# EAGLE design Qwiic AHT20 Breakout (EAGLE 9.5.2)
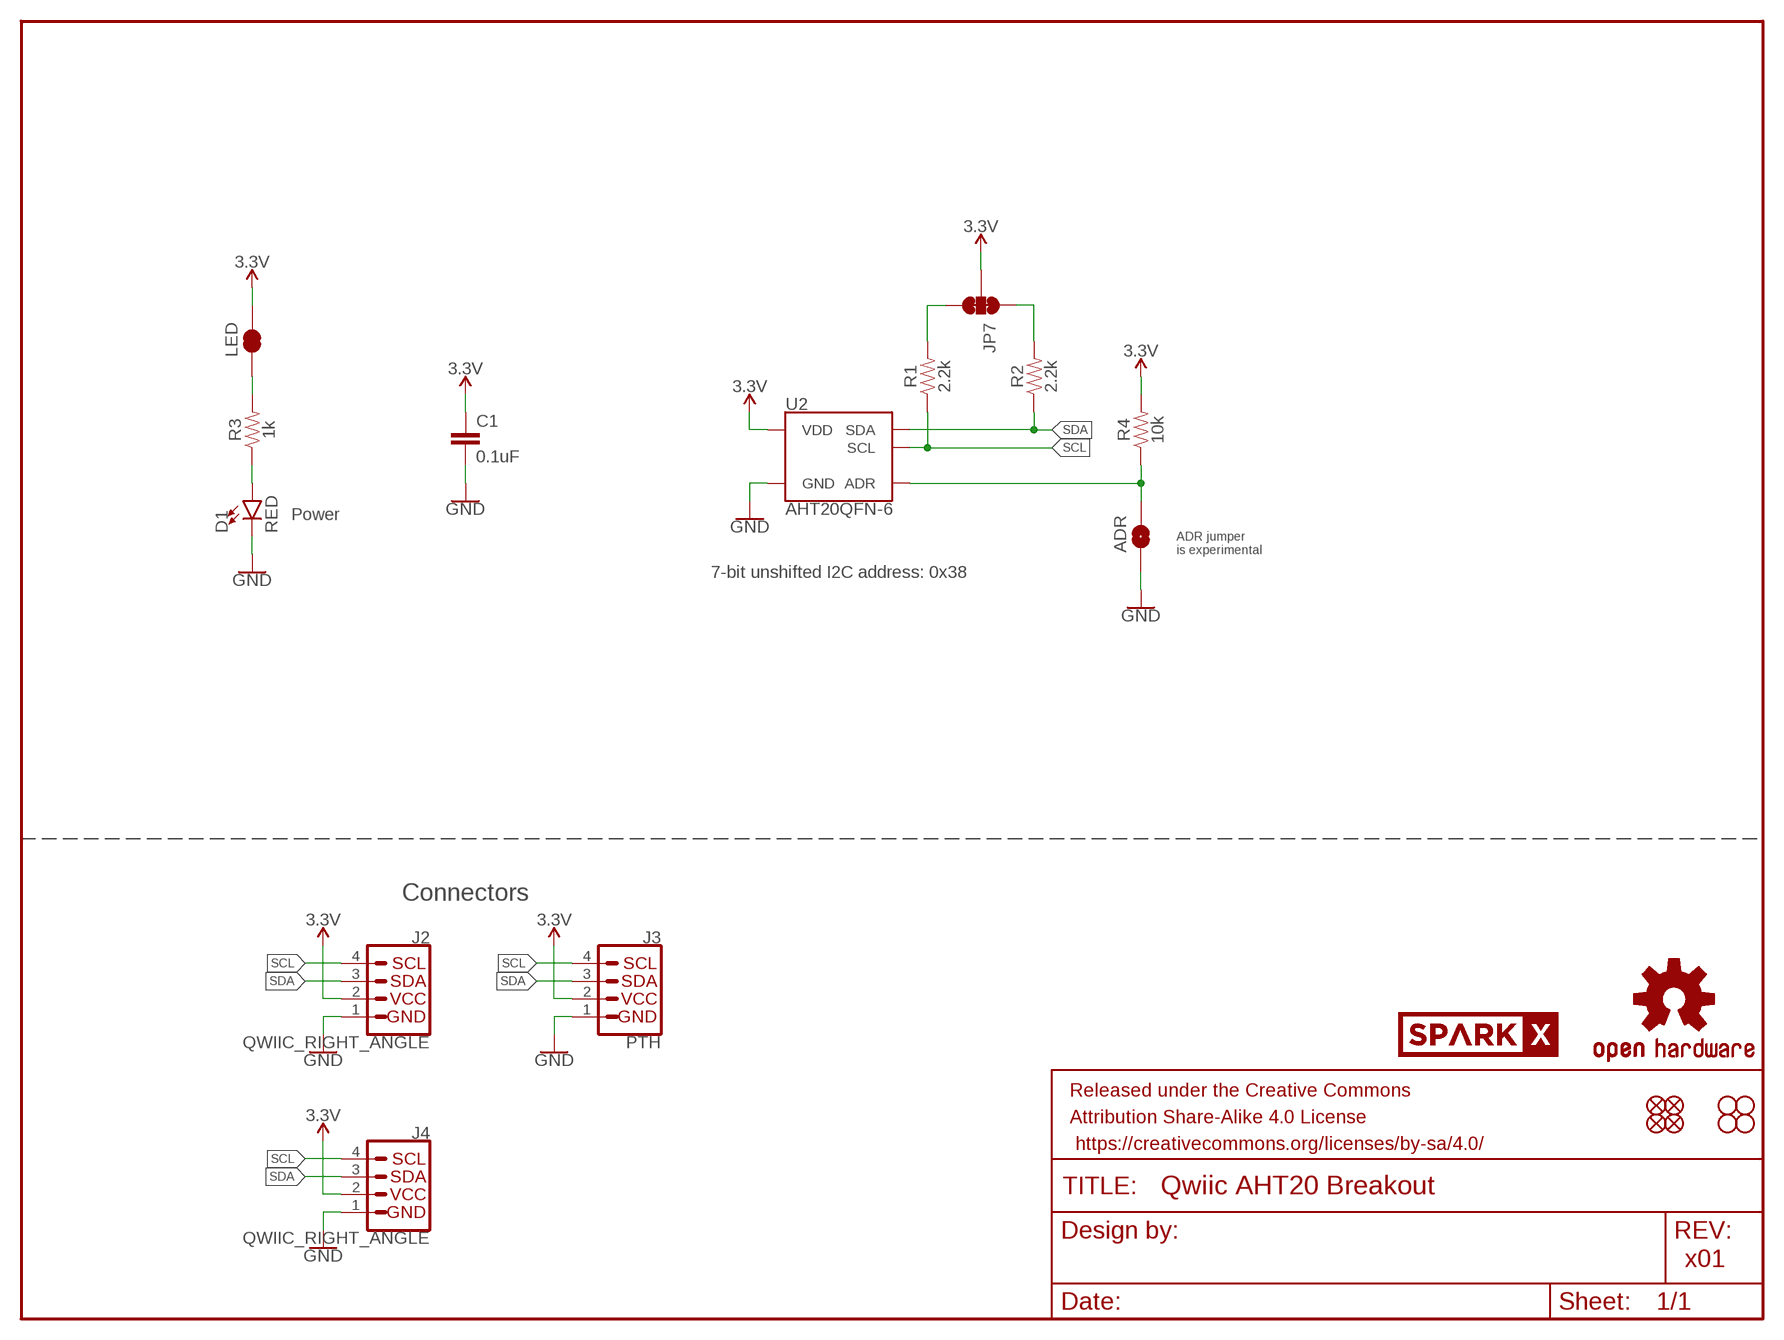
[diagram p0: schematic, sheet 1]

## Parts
ADR  JUMPER-SMT_2_NO_SILK  [SMT-JUMPER_2_NO_SILK]
C1  0.1uF  0.1UF-0603-25V-(+80/-20%)  [0603]
D1  RED  LED-RED0603  [LED-0603]
FRAME1  FRAME-LETTER  [CREATIVE_COMMONS]
J2  QWIIC_RIGHT_ANGLE  QWIIC_CONNECTORJS-1MM  [JST04_1MM_RA]
J3  PTH  I2C_STANDARD_NO_SILK  [1X04_NO_SILK]
J4  QWIIC_RIGHT_ANGLE  QWIIC_CONNECTORJS-1MM  [JST04_1MM_RA]
JP1  FIDUCIAL1X2  [FIDUCIAL-1X2]
JP2  FIDUCIAL1X2  [FIDUCIAL-1X2]
JP3  STAND-OFF  [STAND-OFF]
JP4  STAND-OFF  [STAND-OFF]
JP5  FIDUCIAL1X2  [FIDUCIAL-1X2]
JP6  FIDUCIAL1X2  [FIDUCIAL-1X2]
JP7  JUMPER-SMT_3_2-NC_TRACE_SILK  [SMT-JUMPER_3_2-NC_TRACE_SILK]
JP8  STAND-OFF  [STAND-OFF]
JP9  STAND-OFF  [STAND-OFF]
LED  JUMPER-SMT_2_NC_TRACE_SILK  [SMT-JUMPER_2_NC_TRACE_SILK]
LOGO1  OSHW-LOGOMINI  [OSHW-LOGO-MINI]
R1  2.2k  2.2KOHM-0603-1/10W-1%  [0603]
R2  2.2k  2.2KOHM-0603-1/10W-1%  [0603]
R3  1k  1KOHM-0603-1/10W-1%  [0603]
R4  10k  10KOHM-0603-1/10W-1%  [0603]
U2  AHT20QFN-6  [QFN-6]
U$1  SPARKX-LOGO4  [SPARKX-MEDIUM]
U$2  SPARKX-LOGO4  [SPARKX-MEDIUM]

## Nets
3.3V: C1.1 J2.2 J3.2(VCC) J4.2 JP7.2 LED.2 R4.2 U2.VDD
GND: ADR.1 C1.2 D1.C J2.1 J3.1(GND) J4.1 U2.GND
N$1: JP7.3 R1.2
N$2: JP7.1 R2.2
N$3: D1.A R3.1
N$4: LED.1 R3.2
N$5: ADR.2 R4.1 U2.ADR
SCL: J2.4 J3.4(SCL) J4.4 R1.1 U2.SCL
SDA: J2.3 J3.3(SDA) J4.3 R2.1 U2.SDA

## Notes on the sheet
- Power
- ADR jumper
  is experimental
- 7-bit unshifted I2C address: 0x38
- Connectors
- x01

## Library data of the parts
ADR = SparkFun-Jumpers:JUMPER-SMT_2_NO: Normally open jumper
C1 = SparkFun-Capacitors:0.1UF: 0.1µF ceramic capacitors; PROD_ID: CAP-00810
D1 = SparkFun-LED:LED-RED: Red SMD LED; PROD_ID: DIO-00819
FRAME1 = SparkFun-Aesthetics:FRAME-LETTER: Schematic Frame - Letter
J2 J4 = SparkFun-Connectors:QWIIC_CONNECTOR: SparkFun I2C Standard Qwiic Connector An SMD 1mm pitch JST connector makes it easy and quick (get it? Qwiic?) to connect I2C devices to each other. The Qwiic system enables fast and solderless connection between popular platforms and various sensors and actuators. We carry 200mm, 100mm, 50mm, and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; PROD_ID: CONN-13694
J3 = SparkX:I2C_STANDARD: SparkFun I2C Standard Pinout Header SparkFun has standardized on a pinout for all I2C based sensor breakouts. This pinout allows I2C boards to be plugged directly into the headers on Arduino Uno compatible boards, and to be daisy chained easily. Example SparkFun Products: SparkFun Atmospheric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
JP1 JP2 JP5 JP6 = SparkFun-Aesthetics:FIDUCIAL: Fiducial Alignment Points
JP3 JP4 JP8 JP9 = SparkFun-Hardware:STAND-OFF: Stand Off
JP7 = SparkFun-Jumpers:JUMPER-SMT_3_2-NC_TRACE: Normally closed trace jumper (2 of 2 connections) This jumper has a trace between all three pads so they are normally closed (NC). Use a razor knife to open the connection(s). For best results follow the IPC guidelines for cutting traces: Cutout at least 0.063 mm (0.005 in). Remove all loose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
LED = SparkFun-Jumpers:JUMPER-SMT_2_NC_TRACE: Normally closed trace jumper
LOGO1 = SparkFun-Aesthetics:OSHW-LOGO: Open-Source Hardware (OSHW) Logo
R1 R2 = SparkFun-Resistors:2.2KOHM: 2.2kΩ resistor; PROD_ID: RES-08272
R3 = SparkFun-Resistors:1KOHM: 1kΩ resistor; PROD_ID: RES-07856
R4 = SparkFun-Resistors:10KOHM: 10kΩ resistor; PROD_ID: RES-00824
U2 = AHT20:AHT20: Aosong AHT20 I2C Humidity and Temperature Sensor The AHT20 is a low-cost, easy-to-use, highly accurate, digital humidity and temperature sensor. AHT20 is equipped with a newly designed ASIC chip, an improved MEMS semiconductor capacitive humidity sensing element and a standard on-chip temperature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; PROD_ID: IC-
U$1 U$2 = SparkX:SPARKX-LOGO

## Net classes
1 power: width 0.203 mm

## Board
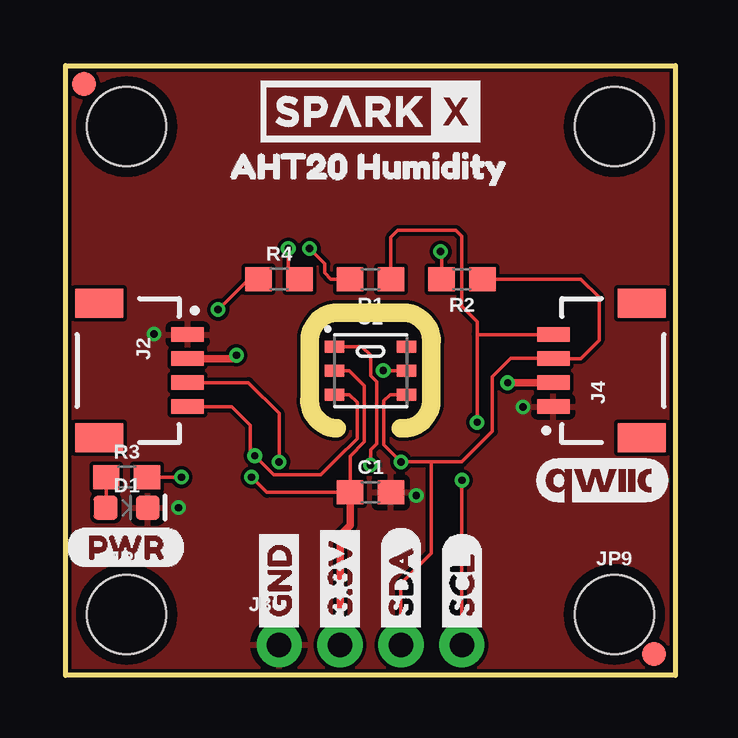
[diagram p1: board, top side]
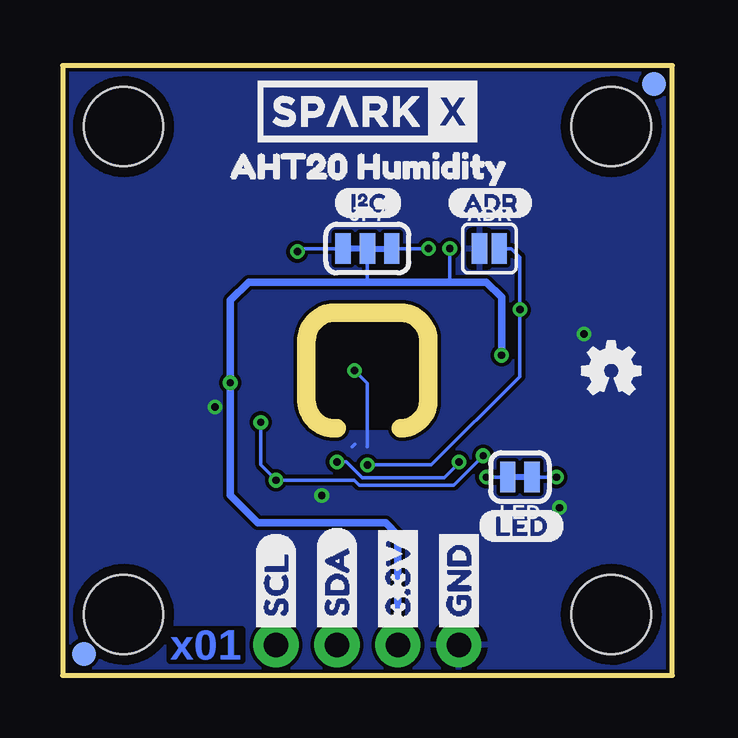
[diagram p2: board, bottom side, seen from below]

Size 25.4 x 25.4 mm. Coordinates in mm from the lower left corner, seen from the top.
Outline: 13.97,10.29 arc92 15.24,11.43 15.24,13.84 arc92 14.1,15.11 11.43,15.11 arc92 10.16,13.97 10.16,11.56 arc92 11.3,10.29
Outline: 0,0 0,25.4 25.4,25.4 25.4,0 0,0
Copper layers (1*16): Top 0.035mm / dielectric 1.5mm / Bottom 0.035mm
Design rules "SparkFun-2-layer-PCBWay-LIMIT": minimum track width 6mil, minimum drill 0.3mm, track to track 6mil, track to pad 6mil, pad to pad 6mil, via to via 6mil, smd to smd 6mil, copper to edge 6mil, drill to drill 6mil, minimum pad ring 6mil, minimum via ring 6mil, stop-mask expansion 4mil, vias tented up to drill 25mil, thermal gap 10mil

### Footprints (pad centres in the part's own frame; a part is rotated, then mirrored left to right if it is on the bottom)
SMT-JUMPER_2_NO_SILK = smd 0.635 x 1.27: 1 -0.406,0; 2 0.406,0
0603 = smd 1.1 x 1: 1 -0.85,0; 2 0.85,0
LED-0603 = smd 1 x 1: A -0.877,0; C 0.877,0
JST04_1MM_RA = smd 0.6 x 1.35: 1 -1.5,0; 2 -0.5,0; 3 0.5,0; 4 1.5,0 | smd 1.2 x 2: NC1 2.8,-3.675; NC2 -2.8,-3.675
1X04_NO_SILK = drill 1.016 pad 1.88: 1 0,0; 2 2.54,0; 3 5.08,0; 4 7.62,0
FIDUCIAL-1X2 = smd 1 x 1: 1 0,0
STAND-OFF = hole 3.302: 0,0
SMT-JUMPER_3_2-NC_TRACE_SILK = smd 0.635 x 1.27: 1 -1.016,0; 2 0,0; 3 1.016,0
SMT-JUMPER_2_NC_TRACE_SILK = smd 0.635 x 1.27: 1 -0.508,0; 2 0.508,0
QFN-6 = smd 0.8 x 0.5: ADR -1.5,1; GND 1.5,0; NC2 1.5,1; SCL -1.5,-1; SDA 1.5,-1; VDD -1.5,0

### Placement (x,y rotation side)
ADR  7.62,17.78 0 bottom
C1  12.7,7.62 0 top
D1  2.54,6.99 0 top
FRAME1  not placed on the board
J2  5.08,12.7 270 top
J3  8.89,1.27 0 top
J4  20.32,12.7 90 top
JP1  0.76,24.64 0 bottom
JP2  24.51,0.89 0 top
JP3  2.54,22.86 0 top
JP4  22.86,22.86 0 top
JP5  24.51,0.89 0 bottom
JP6  0.76,24.64 0 top
JP7  12.7,17.78 0 bottom
JP8  2.54,2.54 0 top
JP9  22.86,2.54 0 top
LED  6.35,8.26 180 bottom
LOGO1  2.54,12.7 0 bottom
R1  12.7,16.51 180 top
R2  16.51,16.51 180 top
R3  2.54,8.26 0 top
R4  8.89,16.51 0 top
U2  12.7,12.7 0 top
U$1  12.7,23.5 0 top
U$2  12.7,23.5 0 bottom
U$3  [GND1]  8.89,1.52 90 bottom
U$4  [3#3V2]  11.43,1.52 90 bottom
U$5  [SDA8]  13.97,1.52 90 bottom
U$6  [SCL9]  16.51,1.52 90 bottom
U$8  [AHT20_HUMIDITY2]  19.3,21.21 0 bottom
U$9  [I_SUPER2_C-()-03]  14.1,19.68 0 bottom
U$10  [(PWR)]  0,5.33 0 top
U$11  [QWIIC_5.5MM]  22.35,8.13 0 top
U$12  [LED_32]  8.13,6.22 0 bottom
U$13  [ADR-()-03]  9.4,19.68 0 bottom
U$14  [AHT20_HUMIDITY2]  5.97,21.21 0 top
U$18  [ORDERING_INSTRUCTIONS]  not placed on the board
U$21  [3#3V2]  11.43,1.52 90 top
U$22  [GND1]  8.89,1.52 90 top
U$26  [SCL9]  16.51,1.52 90 top
U$27  [SDA8]  13.97,1.52 90 top

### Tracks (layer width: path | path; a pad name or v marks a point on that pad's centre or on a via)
3.3V  (via drill 0.3)
  Top 0.152: U2.VDD 11.81,12.7 12.45,12.06 12.45,9.73 11.85,9.13 C1.1 8.38,7.62 v7.75,8.26 | R4.2 9.27,16.98 v9.27,17.78
  Top 0.305: J2.2 6.98,13.2 v7.11,13.34 | v18.41,12.19 J4.2 | J3.2 11.43,5.84 11.85,6.26 C1.1
  Bottom 0.152: LED.2 v7.75,8.26 | JP7.2 12.7,16.38 | v9.27,17.78 9.27,16.38
  Bottom 0.305: v7.11,13.34 7.11,15.75 7.75,16.38 9.27,16.38 12.7,16.38 17.65,16.38 18.41,15.62 v18.41,12.19 18.41,7.49 17.27,6.35 11.94,6.35 11.43,5.84 J3.2
GND  (via drill 0.3)
  Top 0.152: U2.GND v13.23,12.7
  Bottom 0.152: 13.23,9.63 13.34,9.53 | v13.23,12.7 12.7,12.17 12.7,9.53
  other vias: 14.61,7.49 19.05,11.18 4.7,6.99 3.68,14.22
  pour Bottom (isolate 0.152): 0,0 0,25.4 25.4,25.4 25.4,0
  pour Top (isolate 0.152): 0,0 0,25.4 25.4,25.4 25.4,0
N$1  (via drill 0.3)
  Top 0.152: R1.2 11.05,16.51 10.79,16.76 10.79,17.14 v10.16,17.78
  Bottom 0.152: JP7.3 v10.16,17.78
N$2  (via drill 0.3)
  Top 0.152: v15.62,17.65 15.66,17.61 R2.2
  Bottom 0.152: JP7.1 15.49,17.78 v15.62,17.65
N$3
  Top 0.152: R3.1 1.69,7.01 D1.A
N$4  (via drill 0.3)
  Top 0.152: R3.2 v4.83,8.26
  Bottom 0.152: LED.1 v4.83,8.26
N$5  (via drill 0.3)
  Top 0.152: U2.ADR 12.34,13.7 12.7,13.34 12.7,12.48 12.95,12.22 12.95,9.65 12.7,9.4 v12.7,8.76 | R4.1 7.62,16.51 v6.35,15.24
  Bottom 0.152: v12.7,8.76 10.03,8.76 6.35,12.45 v6.35,15.24 6.35,17.42 6.71,17.78 ADR.2
N$6
  cutout Bottom (isolate 0.305): 10.41,14.86 14.99,14.86 14.99,10.29 10.41,10.29
  cutout Top (isolate 0.305): 14.99,14.86 10.41,14.86 10.41,10.29 14.99,10.29
SCL  (via drill 0.3)
  Top 0.152: U2.SCL 11.82,11.7 12.14,11.38 12.14,9.86 11.3,9.02 11.29,9.02 10.63,8.36 8.67,8.36 v7.88,9.15 7.7,9.33 7.7,10.41 6.91,11.2 J2.4 | 17.14,14.22 17.14,14.73 16.51,15.37 16.51,18.29 16.26,18.54 13.84,18.54 13.55,18.25 R1.1 | 17.14,14.22 v17.14,10.54 | 17.14,14.22 17.17,14.2 J4.4 | J3.4 v16.51,8.13
  Bottom 0.152: v17.14,10.54 17.14,8.76 v16.51,8.13 13.25,8.13 13.05,7.92 9.1,7.92 v7.88,9.15
SDA  (via drill 0.3)
  Top 0.152: J2.3 7.61,12.2 8.89,10.92 v8.89,8.89 | 15.24,8.89 v13.97,8.89 13.26,9.6 13.26,9.65 13.26,10.16 13.26,11.43 13.53,11.7 U2.SDA | 15.24,8.89 16.51,8.89 17.78,10.16 17.78,12.45 18.54,13.21 J4.3 21.45,13.2 22.23,13.97 22.23,15.75 21.46,16.51 R2.1 | J3.3 13.97,3.81 15.24,5.08 15.24,8.89
  Bottom 0.152: v13.97,8.89 13.58,8.89 12.92,8.23 9.5,8.23 8.89,8.84 v8.89,8.89

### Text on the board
Bottom: x01
Measures: Dimensions in inches
tDocu: 0.8mm board

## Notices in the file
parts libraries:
SparkFun-Resistors: Licensing: Creative Commons ShareAlike 4.0 International - https://creativecommons.org/licenses/by-sa/4.0
SparkFun-Aesthetics: Released under the Creative Commons Attribution Share-Alike 4.0 License
SparkFun-Aesthetics: https://creativecommons.org/licenses/by-sa/4.0
